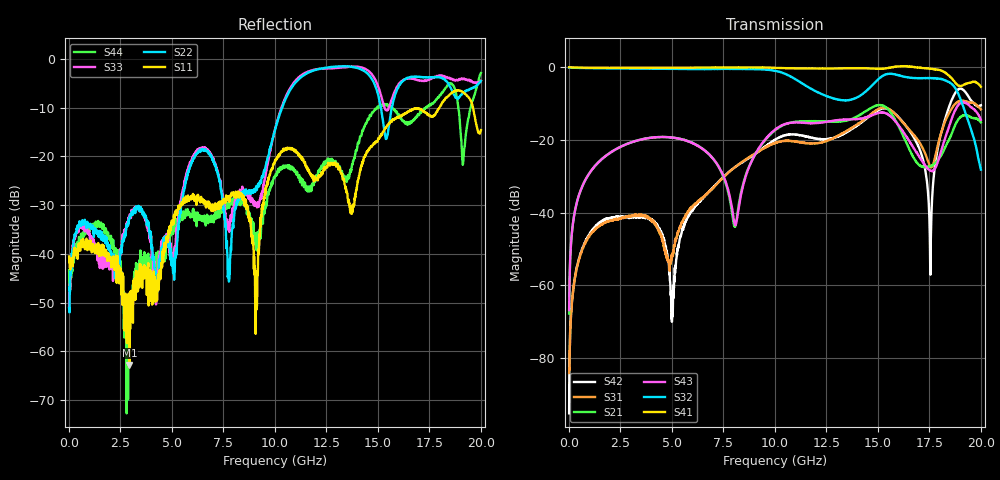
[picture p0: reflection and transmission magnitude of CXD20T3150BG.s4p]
!Keysight Technologies,E5080B,MY59205019,A.15.65.19
!Date: Sunday, June 02, 2024 17:36:22
!Correction: S11(C  4-Port  )
!S12(C  4-Port  )
!S13(C  4-Port  )
!S14(C  4-Port  )
!S21(C  4-Port  )
!S22(C  4-Port  )
!S23(C  4-Port  )
!S24(C  4-Port  )
!S31(C  4-Port  )
!S32(C  4-Port  )
!S33(C  4-Port  )
!S34(C  4-Port  )
!S41(C  4-Port  )
!S42(C  4-Port  )
!S43(C  4-Port  )
!S44(C  4-Port  )
!S4P File: Measurements: <S11,S12,S13,S14>,
!<S21,S22,S23,S24>,
!<S31,S32,S33,S34>,
!<S41,S42,S43,S44>:
# Hz S  dB  R 50
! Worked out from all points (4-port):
!   2000 points, 10 MHz to 20 GHz, reference 50 ohm
!   strongest paths, dB at 10 MHz, 5.01 GHz, 10.01 GHz, 15.01 GHz, 20 GHz:
!     S41: 0.0, -0.1, -0.2, -0.4, -5.4
!     S32: -0.1, -0.4, -1.0, -3.3, -28.1
!     S43: -66.8, -19.4, -17.2, -12.6, -14.4
!     S21: -67.8, -19.3, -17.4, -10.4, -15.2
!     S31: -84.2, -52.3, -20.9, -11.5, -11.6
!     S42: -95.2, -69.2, -20.0, -11.8, -10.4
!   lowest |S11| = -62.8 dB at 2.94 GHz (marker M1), VSWR 1.00, Z = 50.1 - j0.0304 ohm
!   |S11| at or under -10 dB: start of sweep to 17.99 GHz; 19.62 GHz to end of sweep
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1e7  -40.51 159.8  -68.11 83.7  -84.76 104.7  -0.01 -0.1
     -67.79 90.1  -51.11 110.8  -0.05 -0.4  -85.37 137.6
     -84.18 132.2  -0.07 -0.3  -50.83 150.4  -68.21 87.0
     -0.01 -0.2  -95.23 121.7  -66.82 87.5  -43.27 160.8
2.94e9  -62.77 -24.7  -20.81 40.4  -40.97 41.9  -0.15 -14.2
        -20.84 40.5  -32.67 -1.5  -0.36 -83.9  -41.22 40.8
        -40.93 41.6  -0.35 -84.2  -32.75 -13.5  -20.86 40.6
        -0.16 -14.6  -41.16 40.8  -20.86 40.4  -57.19 -132.8
5.02e9  -33.45 172.4  -19.35 2.8  -51.23 -145.1  -0.13 -23.4
        -19.36 2.7  -42.52 -176.3  -0.44 -151.9  -70.23 -122.4
        -51.16 -144.4  -0.45 -152.5  -41.51 169.3  -19.35 3.0
        -0.13 -24.1  -68.14 -119.0  -19.36 2.8  -35.90 -39.5
8.08e9  -27.69 -50.6  -43.65 35.6  -27.37 114.8  -0.02 -43.0
        -43.70 35.3  -30.89 -13.5  -0.47 96.3  -27.38 114.8
        -27.38 113.6  -0.45 95.1  -28.85 -12.8  -43.45 23.3
        -0.06 -44.2  -27.40 113.6  -43.34 23.6  -28.89 142.0
1.545e10  -13.75 150.3  -11.32 -82.3  -11.25 95.0  -0.23 -96.2
          -11.30 -82.0  -15.75 125.3  -1.88 105.2  -11.43 107.4
          -11.24 92.9  -1.88 103.0  -10.48 123.3  -12.84 -70.3
          -0.25 -98.5  -11.42 104.8  -12.86 -70.6  -9.32 -129.0
1.754e10  -11.78 154.0  -27.24 -127.5  -27.29 94.1  -0.38 -117.3
          -27.24 -127.3  -3.76 119.2  -2.97 23.3  -54.99 100.1
          -27.32 91.2  -2.99 20.6  -4.12 99.1  -28.46 -171.2
          -0.42 -120.2  -55.54 89.7  -28.46 -171.0  -9.36 131.9
2e10  -14.61 2.5  -15.17 -27.6  -11.63 37.2  -5.35 140.3
      -15.17 -27.7  -4.54 44.4  -28.18 -79.6  -10.43 87.8
      -11.61 33.7  -28.15 -82.7  -4.48 62.7  -14.38 -4.5
      -5.36 136.9  -10.43 84.4  -14.45 -4.7  -2.90 -56.8
